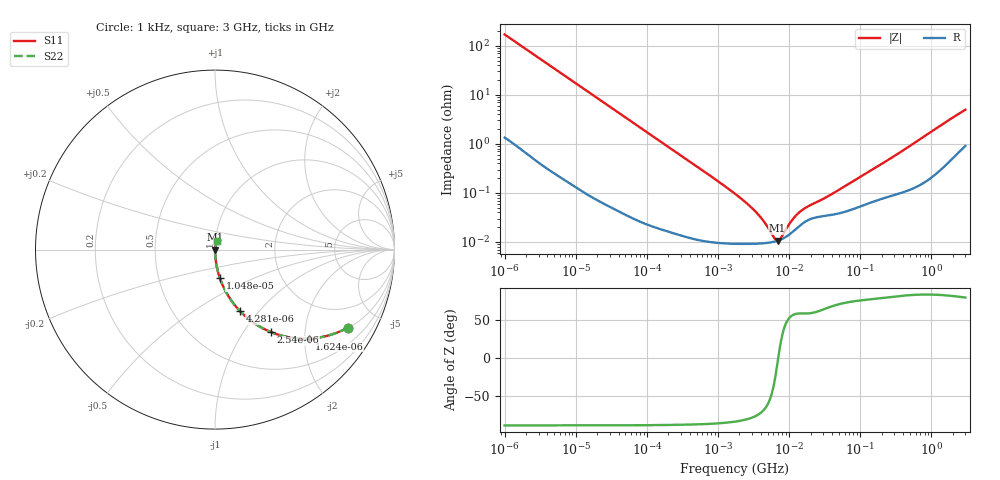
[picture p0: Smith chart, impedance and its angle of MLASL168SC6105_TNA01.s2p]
! MLASL168SC6105_TNA01  S-PARAMETER MODEL  ( Standard Model )
! Model Generated by TAIYO YUDEN Corporation (http://www.ty-top.com)
! Version 1.0
! TAIYO YUDEN Control No. 220601
! Copyright(c) 2012 TAIYO YUDEN CO.,LTD. All Rights Reserved.
! Product Description (link to TY-COMPAS)
! https://ds.yuden.co.jp/TYCOMPAS/or/detail?pn=MLASL168SC6105KTNA01&u=M
! Products Name : Multilayer Ceramic Capacitors
! Characteristics :
!  Capacitance : 1 [uF] , Rated Voltage : 10 [V] , TCC : X6S
!  Case Size : 1.6 x 0.8 / 0.063 x 0.031 [mm/inch] , Thickness : 0.8 / 0.031 [mm/inch]
!  (Conditions: Temperature = 25 [degC] , DC Bias Voltage = 0 [V])
! External Node Assignments :
!  1  o---| |---o  2
! GND o---------o GND
! Frequency Range : 1kHz  -  3GHz  [ 401 STEP ]
# MHZ S RI R 50
! Freq[MHz].  S11 Real  S11 Imag  S21 Real  S21 Imag  S12 Real  S12 Imag  S22 Real  S22 Imag
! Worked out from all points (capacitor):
!   401 points, 1 kHz to 3 GHz, reference 50 ohm
!   read as one part in series: C = 935 nF near 1.077 kHz
!   lowest |Z| = 10.7 mohm at 6.882 MHz (marker M1)
!   series resonance near 7.026 MHz, so ESL is about 550 pH
!   S11 on the Smith chart (normalised r, x): 1 kHz: 1.03, -3.40; 1.624 kHz: 1.02, -2.10; 2.54 kHz: 1.01, -1.35; 4.281 kHz: 1.01, -0.80; 10.47 kHz: 1.00, -0.33; 3 GHz: 1.02, +0.10
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0.001  0.7412 -0.4341  0.2588 0.4341  0.2588 0.4341  0.7412 -0.4341
0.001624  0.5241 -0.4956  0.4759 0.4956  0.4759 0.4956  0.5241 -0.4956
0.00254  0.3128 -0.46  0.6872 0.46  0.6872 0.46  0.3128 -0.46
0.004281  0.1397 -0.3431  0.8603 0.3431  0.8603 0.3431  0.1397 -0.3431
0.006451  0.0676 -0.2474  0.9324 0.2474  0.9324 0.2474  0.0676 -0.2474
0.010475  0.0274 -0.1594  0.9726 0.1594  0.9726 0.1594  0.0274 -0.1594
0.01216  0.0206 -0.1384  0.9794 0.1384  0.9794 0.1384  0.0206 -0.1384
0.033275  0.00317 -0.0517  0.9968 0.0517  0.9968 0.0517  0.00317 -0.0517
0.147855  0.000325 -0.0118  0.9997 0.0118  0.9997 0.0118  0.000325 -0.0118
1.732051  9.26e-05 -0.000956  0.9999 0.000956  0.9999 0.000956  9.26e-05 -0.000956
3.517417  9.23e-05 -0.000378  0.9999 0.000378  0.9999 0.000378  9.23e-05 -0.000378
4.566395  9.46e-05 -0.000226  0.9999 0.000226  0.9999 0.000226  9.46e-05 -0.000226
6.153411  0.000101 -6.79e-05  0.9999 6.79e-05  0.9999 6.79e-05  0.000101 -6.79e-05
6.881678  0.000106 -1.06e-05  0.9999 1.06e-05  0.9999 1.06e-05  0.000106 -1.06e-05
7.696136  0.000113 4.68e-05  0.9999 -4.68e-05  0.9999 -4.68e-05  0.000113 4.68e-05
10.37087  0.000147 0.000201  0.9999 -0.000201  0.9999 -0.000201  0.000147 0.000201
12.49624  0.000184 0.000294  0.9998 -0.000294  0.9998 -0.000294  0.000184 0.000294
15.62917  0.000241 0.000392  0.9998 -0.000392  0.9998 -0.000392  0.000241 0.000392
21.06097  0.000301 0.000504  0.9997 -0.000504  0.9997 -0.000504  0.000301 0.000504
41.2049  0.000361 0.000905  0.9996 -0.000905  0.9996 -0.000905  0.000361 0.000905
256.0921  0.000866 0.0048  0.9991 -0.0048  0.9991 -0.0048  0.000866 0.0048
3000  0.0113 0.0479  0.9887 -0.0479  0.9887 -0.0479  0.0113 0.0479
